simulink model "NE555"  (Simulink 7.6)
settings: Solver=ode15s  StartTime=0.0  StopTime=10.0  RelTol=1e-3
libraries: elec_lib x6, fl_lib x3

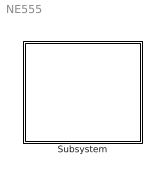
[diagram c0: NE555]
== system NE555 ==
  Subsystem : Subsystem

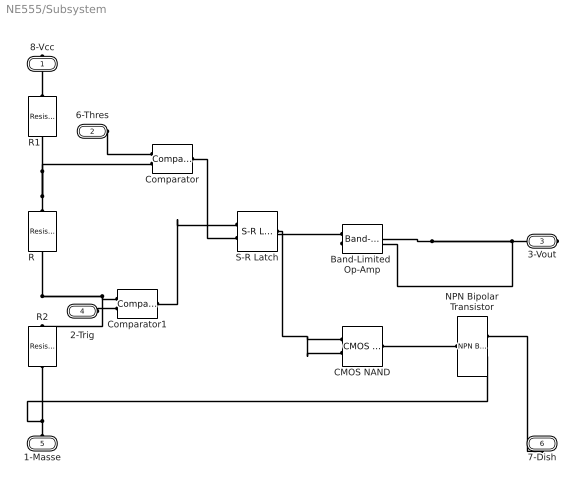
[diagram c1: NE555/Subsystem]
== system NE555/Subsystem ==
  Band-Limited  Op-Amp : elec_lib/Integrated Circuits/Band-Limited Op-Amp  DialogController=NetworkEngine.DynNeDlgSource  SystemSampleTime=-1  A=1000  Rin=1e+6 Ohm  Rout=100 Ohm  Vmin=-15 V  Vmax=15 V  Vdotmax=1000 V/s  f=1e+5 Hz  V0=0 V  LocalVarLogging=[]
  CMOS NAND : elec_lib/Integrated Circuits/Logic/CMOS NAND  DialogController=NetworkEngine.DynNeDlgSource  SystemSampleTime=-1  V_IL=2 V  V_IH=3 V  C_IN=5 pF  output_type=1  V_OL=0 V  V_OH=5 V  V_CC=5 V  V_meas=5 V  R_OUT=25 Ohm  R_OH=[ 25 250 ] Ohm  I_OH=63 mA  R_OL=[ 30 800 ] Ohm  I_OL=-45 mA  Delay=25 ns  Ron=5 Ohm  Vf=0.6 V  output_state=1  LocalVarLogging=[]
  Comparator : elec_lib/Integrated Circuits/Comparator  DialogController=NetworkEngine.DynNeDlgSource  SystemSampleTime=-1  V_OS=5 mV  V_OL=0 V  V_OH=5 V  C_IN=0 pF  R_OUT=50 Ohm  Delay=0 s  LocalVarLogging=[]
  Comparator1 : elec_lib/Integrated Circuits/Comparator  DialogController=NetworkEngine.DynNeDlgSource  SystemSampleTime=-1  V_OS=5 mV  V_OL=0 V  V_OH=5 V  C_IN=0 pF  R_OUT=50 Ohm  Delay=0 s  LocalVarLogging=[]
  NPN Bipolar Transistor : elec_lib/Semiconductor Devices/NPN Bipolar Transistor  DialogController=NetworkEngine.DynNeDlgSource  SystemSampleTime=-1  parameterization=1  BF=100  IS=1e-14 A  VAF=200 V  hfe=100  hoe=5e-5 1/Ohm  Ic_h=1 mA  V1=0.55 V  I1=0.5 mA  BR=1  Tmeas=25 C  RC=0.01 Ohm  RE=1e-4 Ohm  RB=1 Ohm  C_BC=5 pF  C_BE=5 pF  TF=0 us  TR=0 us  LocalVarLogging=[]
  R : fl_lib/Electrical/Electrical Elements/Resistor  DialogController=NetworkEngine.DynNeDlgSource  SystemSampleTime=-1  R=5 kOhm  i_Log=off  v_Log=off  LocalVarNames=|current|voltage|power  LocalVarDescs=|Resistor current (A)|Voltage across resistor (V)|Power (W)  LocalVarLogging=[0 0 0]
  R1 : fl_lib/Electrical/Electrical Elements/Resistor  DialogController=NetworkEngine.DynNeDlgSource  SystemSampleTime=-1  R=5 kOhm  i_Log=off  v_Log=off  LocalVarNames=|current|voltage|power  LocalVarDescs=|Resistor current (A)|Voltage across resistor (V)|Power (W)  LocalVarLogging=[0 0 0]
  R2 : fl_lib/Electrical/Electrical Elements/Resistor  DialogController=NetworkEngine.DynNeDlgSource  SystemSampleTime=-1  R=5 kOhm  i_Log=off  v_Log=off  LocalVarNames=|current|voltage|power  LocalVarDescs=|Resistor current (A)|Voltage across resistor (V)|Power (W)  LocalVarLogging=[0 0 0]
  S-R Latch : elec_lib/Integrated Circuits/Logic/S-R Latch  DialogController=NetworkEngine.DynNeDlgSource  SystemSampleTime=-1  V_IL=2 V  V_IH=3 V  C_IN=5 pF  output_type=1  V_OL=0 V  V_OH=5 V  V_CC=5 V  V_meas=5 V  R_OUT=25 Ohm  R_OH=[ 25 250 ] Ohm  I_OH=63 mA  R_OL=[ 30 800 ] Ohm  I_OL=-45 mA  Delay=25 ns  Ron=5 Ohm  Vf=0.6 V  output_state=1  LocalVarLogging=[]
  8-Vcc : PMIOPort  Port=1  Side=Right
  6-Thres : PMIOPort  Port=2  Side=Left
  3-Vout : PMIOPort  Port=3  Side=Right
  2-Trig : PMIOPort  Port=4  Side=Left
  1-Masse : PMIOPort  Port=5  Side=Left
  7-Dish : PMIOPort  Port=6  Side=Right
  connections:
  S-R Latch/RConn1 -- Band-Limited  Op-Amp/LConn1 -- CMOS NAND/LConn1 -- CMOS NAND/LConn2
  3-Vout/RConn1 -- Band-Limited  Op-Amp/RConn1 -- Band-Limited  Op-Amp/LConn2
  R/LConn1 -- Comparator/LConn2 -- R1/RConn1
  Comparator/RConn1 -- S-R Latch/LConn2
  Comparator1/LConn1 -- R/RConn1 -- R2/LConn1
  Comparator1/RConn1 -- S-R Latch/LConn1
  8-Vcc/RConn1 -- R1/LConn1
  6-Thres/RConn1 -- Comparator/LConn1
  2-Trig/RConn1 -- Comparator1/LConn2
  1-Masse/RConn1 -- R2/RConn1 -- NPN Bipolar Transistor/RConn2
  CMOS NAND/RConn1 -- NPN Bipolar Transistor/LConn1
  NPN Bipolar Transistor/RConn1 -- 7-Dish/RConn1
